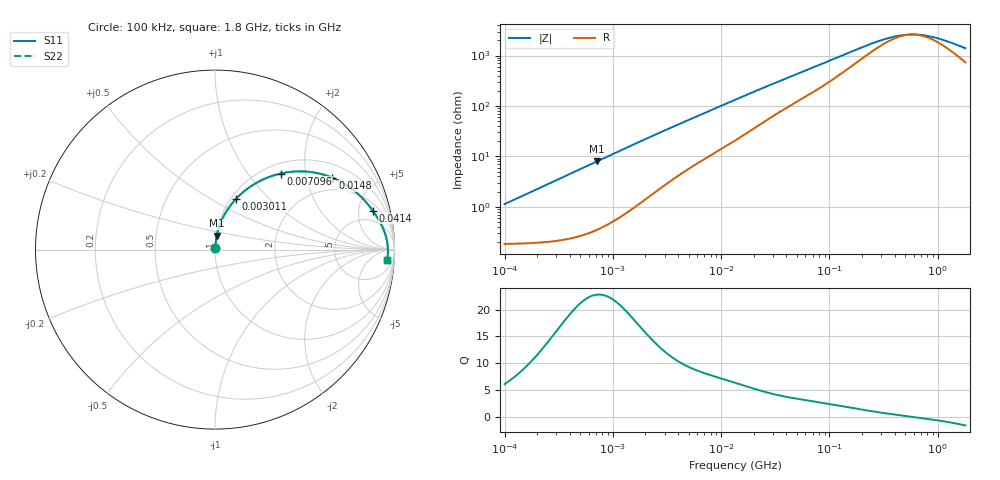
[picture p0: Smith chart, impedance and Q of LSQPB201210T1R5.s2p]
! LSQPB201210T1R5  S-PARAMETER MODEL  ( General Type )
! Model Generated by TAIYO YUDEN Corporation (http://www.ty-top.com)
! Version 2.0
! TAIYO YUDEN Control No. 100810NF18SB-HKC
! Copyright(c) 2007 TAIYO YUDEN CO.,LTD. All Rights Reserved.
! Product Description (link to TY-COMPAS)
! https://ds.yuden.co.jp/TYCOMPAS/or/detail?pn=LSQPB201210T1R5M&u=M
! Products Name : Inductors
! Characteristics :
!  Inductance : 1.5 uH , SRF(min) : 250 MHz , DC Resistance(max) : 0.234 Ohm
!  Rated Current : Saturation :700 mA , Temp Rise : 750 mA (40 degC)
!  Case Size : 2.0 x 1.25 / 0.079 x 0.049 [mm/inch] , Thickness : 1.0 / 0.04 [mm/inch]
!  (Conditions: Temperature = 25 degC , DC Bias Current/Voltage = 0A / 0V)
! External Node Assignments :
!  1  o---GGG---o  2
! GND o---------o GND
! Frequency Range : 0.1MHz  -  1800MHz  [ 402 STEP ]
# MHz S RI R 50
! Freq[MHz].  S11 Real  S11 Imag  S21 Real  S21 Imag  S12 Real  S12 Imag  S22 Real  S22 Imag
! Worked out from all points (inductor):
!   401 points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, 100 kHz to 1.8 GHz, reference 50 ohm
!   read as one part in series: L = 1.78 uH near 105 kHz
!   highest Q = 22.8 at 709.7 kHz (marker M1), where L = 1.78 uH
!   self-resonance near 578.4 MHz
!   S11 on the Smith chart (normalised r, x): 100 kHz: 1.00, +0.02; 3.011 MHz: 1.05, +0.65; 7.096 MHz: 1.18, +1.45; 14.8 MHz: 1.47, +2.86; 41.4 MHz: 2.91, +7.01; 1.8 GHz: 16, -24
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0.1  0.00195 0.0111  0.998 -0.0111  0.998 -0.0111  0.00195 0.0111
0.253659  0.00281 0.0282  0.9972 -0.0282  0.9972 -0.0282  0.00281 0.0282
0.516129  0.00597 0.0572  0.994 -0.0572  0.994 -0.0572  0.00597 0.0572
0.709667  0.00963 0.0782  0.9904 -0.0782  0.9904 -0.0782  0.00963 0.0782
1.516485  0.0358 0.1606  0.9642 -0.1606  0.9642 -0.1606  0.0358 0.1606
2.66389  0.0948 0.2573  0.9052 -0.2573  0.9052 -0.2573  0.0948 0.2573
3.010975  0.1156 0.2812  0.8844 -0.2812  0.8844 -0.2812  0.1156 0.2812
4.566214  0.214 0.3618  0.786 -0.3618  0.786 -0.3618  0.214 0.3618
7.096489  0.3649 0.4236  0.6351 -0.4236  0.6351 -0.4236  0.3649 0.4236
9.75753  0.4933 0.4355  0.5067 -0.4355  0.5067 -0.4355  0.4933 0.4355
13.41641  0.6191 0.4134  0.3809 -0.4134  0.3809 -0.4134  0.6191 0.4134
14.79752  0.6544 0.4005  0.3456 -0.4005  0.3456 -0.4005  0.6544 0.4005
24.15197  0.7927 0.3138  0.2073 -0.3138  0.2073 -0.3138  0.7927 0.3138
41.39926  0.8787 0.2174  0.1213 -0.2174  0.1213 -0.2174  0.8787 0.2174
69.24595  0.9231 0.1455  0.0769 -0.1455  0.0769 -0.1455  0.9231 0.1455
121.6389  0.9482 0.0871  0.0518 -0.0871  0.0518 -0.0871  0.9482 0.0871
218.9722  0.959 0.045  0.041 -0.045  0.041 -0.045  0.959 0.045
357.3983  0.9622 0.0201  0.0378 -0.0201  0.0378 -0.0201  0.9622 0.0201
516.0898  0.9631 0.00461  0.0369 -0.00461  0.0369 -0.00461  0.9631 0.00461
727.2099  0.9633 -0.00934  0.0367 0.00934  0.0367 0.00934  0.9633 -0.00934
1050.104  0.9628 -0.0256  0.0372 0.0256  0.0372 0.0256  0.9628 -0.0256
1800  0.9603 -0.0563  0.0397 0.0563  0.0397 0.0563  0.9603 -0.0563
